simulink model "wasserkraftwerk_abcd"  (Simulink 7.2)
settings: Solver=ode23tb  StartTime=0.0  StopTime=1000  MaxStep=0.1  RelTol=1e-3
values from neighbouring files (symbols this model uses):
  x_IC = 0    [Parameter_sim.m]
undefined symbols (not defined in the file or in its folder): A, B, C, D, sigbuilder_block

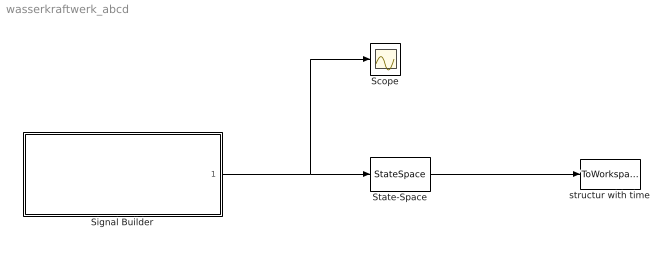
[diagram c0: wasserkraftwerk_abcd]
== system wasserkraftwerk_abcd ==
  Scope : Scope
  Signal Builder : Subsystem  Tag=STV Subsys  LoadFcn=sigbuilder_block('load');  StartFcn=sigbuilder_block('start');  StopFcn=sigbuilder_block('stop');  ClipboardFcn=sigbuilder_block('clipboard');
  State-Space : StateSpace  A=A  B=B  C=C  D=D  X0=x_IC
  structur with time : ToWorkspace  VariableName=abcd  SampleTime=-1  SaveFormat=Structure With Time
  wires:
  State-Space/1 -> structur with time/1
  Signal Builder/1(u) -> State-Space/1, Scope/1

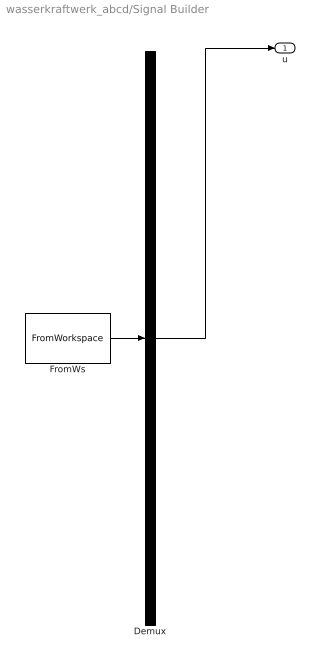
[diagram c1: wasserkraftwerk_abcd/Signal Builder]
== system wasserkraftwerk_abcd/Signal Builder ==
  Demux : Demux  Tag=STV Demux  Outputs=1
  FromWs : FromWorkspace  Tag=STV FromWs  VariableName=tuvar  SampleTime=0  SigBuilderData=DataTag0  VnvData=DataTag1
  u : Outport  Tag=STV Outport  OutDataType=sfix(16)  OutScaling=2^0
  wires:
  Demux/1 -> u/1
  FromWs/1 -> Demux/1
